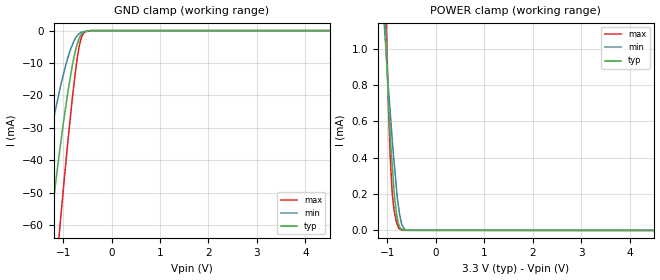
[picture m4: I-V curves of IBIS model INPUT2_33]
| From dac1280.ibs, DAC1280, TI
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|   INPUT2_33   3.3V digital input Model
[Model]   INPUT2_33
Model_type   Input
|  Signals : _PWDN(16)
Vinl = 0.66
Vinh = 2.34
|   typ   min   max
|   (nom PVT)   (Fast PVT)   (slow PVT)
C_comp   2.4535150e-12   1.8399700e-12   3.1435790e-12
| Where   nom PVT is  Nominal Process, 3.3V, 27C
|   Fast PVT is Strong Process, 3.6V, -40C
|   Slow PVT is Weak Process, 3.0V, 85C
[Voltage Range]   3.3   3   3.6
[Temperature Range]   27   85   -40
[Power Clamp Reference]   3.3   3   3.6
[GND Clamp Reference]   0   0   0
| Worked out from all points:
|   GND clamp passes 1 mA (typ) near -0.62 V on its own axis
|   POWER clamp passes 1 mA (typ) near -1.02 V on its own axis
[GND Clamp]
|   Voltage   I(typ)   I(min)   I(max)
-3.3V     -365.5mA   -258.9mA   -460.2mA
-1.597V   -106mA     -62.12mA   -153.3mA
-1.296V   -64.68mA   -35.02mA   -99.72mA
-1.202V   -52.57mA   -27.66mA   -83.32mA
-1.089V   -38.89mA   -19.5mA    -64.05mA
-1.054V   -34.94mA   -17.04mA   -58.12mA
-812mV    -10.83mA   -4.451mA   -21.03mA
-706.7mV  -3.936mA   -1.508mA   -8.155mA
-630.7mV  -1.241mA   -525.7uA   -2.473mA
-554.3mV  -267.8uA   -311.7uA   -396.5uA
-426.7mV  -11.62uA   -13.55uA   -7.152uA
6.6V      0A         0A         0A
[POWER Clamp]
|   Voltage   I(typ)   I(min)   I(max)
-3.3V     30.92mA    25.65mA    38.05mA
-1.057V   1.262mA    1.102mA    1.572mA
-1.022V   988.4uA    952.9uA    1.141mA
-1.015V   943.9uA    924uA      1.063mA
-972.9mV  681.5uA    762.7uA    640.3uA
-942.5mV  532.8uA    652.4uA    408.8uA
-901.3mV  364.2uA    503.2uA    211.4uA
-859.7mV  209.7uA    372.2uA    108.6uA
-812mV    91.53uA    228.1uA    43.91uA
-750.2mV  23.25uA    90.32uA    9.291uA
-689.4mV  5.726uA    26.04uA    922.4nA
6.6V      0A         0A         0A
